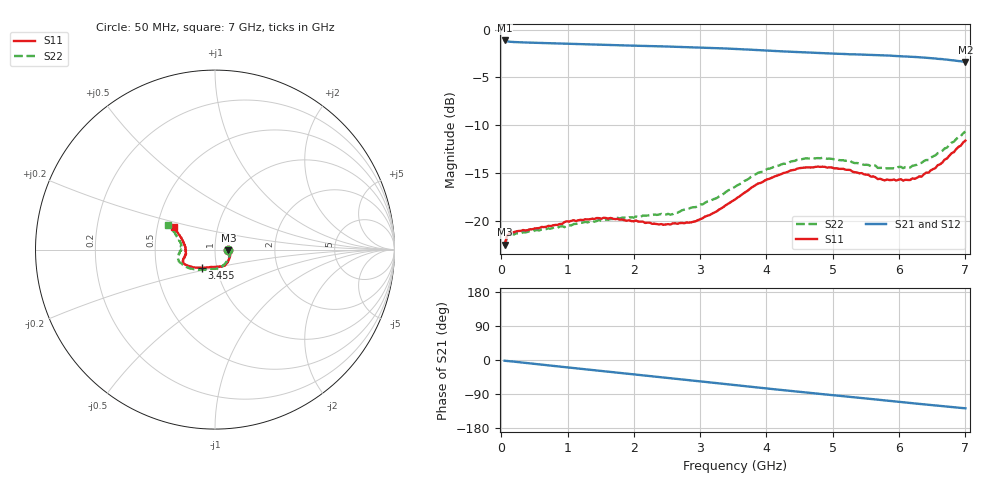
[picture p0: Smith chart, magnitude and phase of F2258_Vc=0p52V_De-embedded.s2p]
! Integrated Device Technology
! Corporate Headquarters
! 6024 Silver Creek Valley Road
! San Jose, CA 95138  USA
! Phone:  1-408-284-8200
! Toll Free:  1-800-223-1366
! Webpage:  http://www.idt.com/
! Timing and RF Division
! 515 Groton Road, Suite 102
! Westford, MA 01886-6024
! Device:  F2258
! Description: Voltage Variable RF Attenuator
! Frequency:  50.0 -  6000.00 MHz
! Package:  3x3 mm Thin QFN Plastic Package: 16 pin
! Ports:  2 RF, 2 DC
!  Pin  1  = NC
!  Pin  2  = NC
!  Pin  3  = RF2  = Port 2
!  Pin  4  = GND
!  Pin  5  = Vdd
!  Pin  6  = NC
!  Pin  7  = VCTRL
!  Pin  8  = NC
!  Pin  9  = GND
!  Pin 10  = RF1  = Port 1
!  Pin 11  = NC
!  Pin 12  = NC
!  Pin 13  = NC
!  Pin 14  = NC
!  Pin 15  = NC
!  Pin 16  = NC
! Vcntrl:  0.520 Volts
! Vdd:  +3.300 Volts
! Current:  1.102 mA
! Data:  The device was measured on a the F2258 evaluation board which has
!  individual transmission lines to the RF pins.  Data was collected
!  using a calibrated network analyzer.  The evaluation board was
!  de-embedded using a TRL calibration technique.
!  The reference plane is the edge of the package pin.
! Misc:  SN 10
!  Action Tracker AT0285
! Date Measured:  2014-12-10
! Date:  2016-01-13  MJV
! Note:
!  Integrated Device Technology supplies this data as a sample of measured
!  data at the package pin for this product.  Your particular data for this
!  product may vary.
!  Data was taken at 25 degrees C.
!  Integrated Device Technology reserves the right to change this data at anytime.
!Freq_(GHz)  S11M_(dB)  S11P_(deg)  S21M_(dB)  S21P_(deg)  S12M_(dB)  S12P_(deg)  S22M_(dB)  S22P_(deg)
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# GHz S dB R 50
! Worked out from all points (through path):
!   201 points, 50 MHz to 7 GHz, reference 50 ohm
!   highest |S21| = -1.13 dB at 50 MHz (marker M1); lowest = -3.4 dB at 7 GHz (marker M2)
!   group delay of S21, straight-line fit = 50.5 ps
!   lowest |S11| = -22.5 dB at 50 MHz (marker M3), VSWR 1.16, Z = 58.1 - j0.455 ohm
!   |S11| at or under -10 dB: start of sweep to end of sweep
!   |S22| runs from -22.7 to -10.7 dB; largest |S21 - S12| = 0.00043
!   S11 on the Smith chart (normalised r, x): 50 MHz: 1.16, -0.01; 3.455 GHz: 0.85, -0.17; 7 GHz: 0.61, +0.16
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0.05  -22.53 -3.0  -1.13 -2.0  -1.13 -2.0  -22.67 -3.0
0.08475  -21.64 -4.8  -1.22 -2.5  -1.22 -2.5  -21.79 -4.9
0.15425  -21.20 -7.6  -1.28 -3.7  -1.28 -3.7  -21.44 -8.4
0.71025  -20.55 -31.3  -1.41 -14.1  -1.41 -14.1  -20.81 -34.9
1.2315  -19.94 -51.2  -1.52 -23.8  -1.52 -23.8  -20.21 -58.5
1.6485  -19.71 -62.1  -1.61 -31.5  -1.61 -31.5  -19.84 -71.6
2.37825  -20.39 -81.2  -1.74 -44.8  -1.74 -44.8  -19.37 -90.1
2.552  -20.40 -86.9  -1.77 -48.0  -1.77 -48.0  -19.37 -95.4
2.93425  -20.06 -103.3  -1.85 -55.1  -1.85 -55.1  -18.58 -109.1
3.247  -19.04 -117.1  -1.93 -61.0  -1.93 -61.0  -17.64 -121.5
3.4555  -18.09 -126.4  -1.99 -64.9  -1.99 -64.9  -16.71 -129.3
3.525  -17.78 -128.9  -2.01 -66.2  -2.01 -66.2  -16.46 -132.3
4.0115  -15.67 -144.6  -2.19 -75.3  -2.19 -75.3  -14.59 -148.4
4.46325  -14.55 -153.9  -2.35 -83.4  -2.35 -83.4  -13.62 -159.9
4.7065  -14.42 -157.2  -2.42 -87.7  -2.43 -87.7  -13.52 -164.3
5.2625  -14.69 -163.9  -2.58 -97.4  -2.58 -97.4  -13.73 -172.6
5.6795  -15.65 -170.0  -2.66 -104.6  -2.66 -104.6  -14.48 -178.3
5.85325  -15.75 -174.2  -2.72 -107.7  -2.72 -107.7  -14.52 177.0
6.166  -15.75 177.8  -2.82 -113.3  -2.82 -113.3  -14.45 170.8
6.33975  -15.39 170.9  -2.90 -116.4  -2.91 -116.4  -13.95 166.4
6.722  -13.49 157.8  -3.13 -123.1  -3.14 -123.1  -12.36 157.2
7  -11.62 151.5  -3.38 -127.4  -3.38 -127.4  -10.66 152.1
